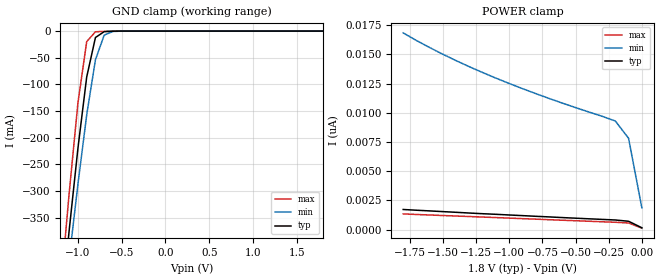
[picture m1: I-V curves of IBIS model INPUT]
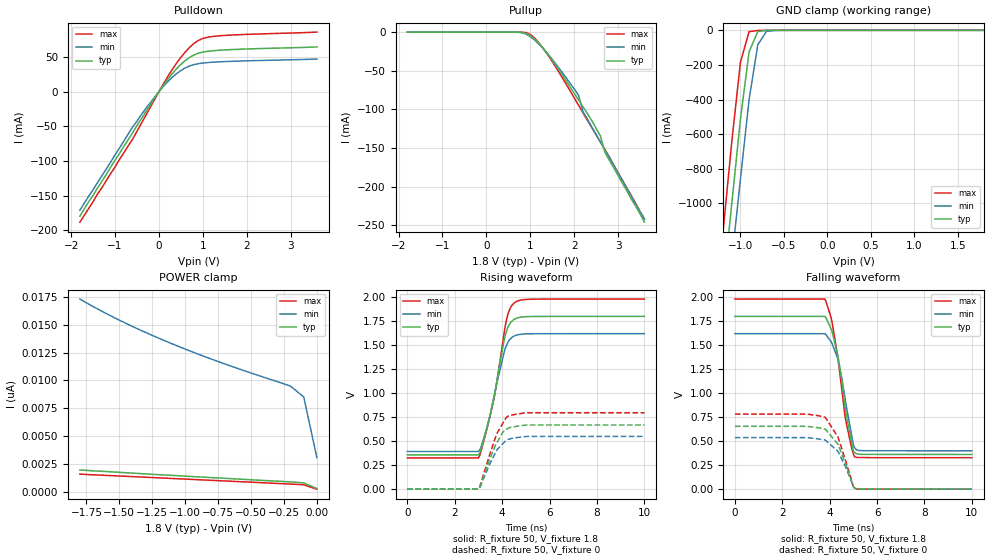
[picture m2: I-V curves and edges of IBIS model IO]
|   PERICOM SEMICONDUCTOR CORP
|   IBIS Model of PI4ULS3V204
|   Product Family: ULS
|   TSSOP-14 (L) Package
[IBIS Ver] 3.2
[Comment char] |_char
[File Name] pi4uls3v204_l_18v.ibs
[File Rev] 1.0
[Source] File originated at Pericom Semiconductor Corp.
[Date] 09/06/2017
[Disclaimer] (C) Copyright PERICOM Semiconductor Corporation
   All rights reserved
  Pericom Semiconductor Corporation hereby grants the user of
  this IBIS model a non-exclusive, nontransferable license to
  use this IBIS model under the following terms.
  This IBIS model is provided on an "AS IS" basis and Pericom
  makes absolutely no warranty with respect to the information
  contained herein. PERICOM DISCLAIMS AND CUSTOMER WAIVES ALL
  WARRANTIES, EXPRESSED OR IMPLIED, INCLUDING WARRANTIES OF
  MERCHANTABILITY OR FITNESS FOR A PARTICULAR PURPOSE. The
  entire risk as to quality and performance is with the customer.
  Accordingly, in no event shall the company be liable for any
  damages, whether in contract or tort, including any lost
  profits or other incidental, consequential, exemplary, or
  punitive damages arising out of the use or application of the
  IBIS model provided in this package. Further, Pericom reserves
  the right to make changes without notice to any product herein
  to improve reliability, function, or design. Pericom does not
  convey any license under patent rights or any other intellectual
  property rights, including those of third parties.
  The user is granted this license only to use the IBIS model
  and is not granted rights to sell, load, rent, lease or license
  the IBIS model in whole or in part, or in modified form to anyone
  other than user. User may modify the IBIS model to suit its specific
  application but rights to derivative works and such modifications
  shall belong to Pericom.
  Pericom is not obligated to provide maintenance or support
  for the licensed IBIS model.
  Contact Pericom at ATTN: APPLICATION ENGINEERING / IBIS MODELS
  1545 Barber Lane Milpitas, CA 95035 USA.
[Component] PI4ULS3V204
[Manufacturer] Pericom Semiconductor Corp.
[Package]
| variable   typ   min   max
R_pkg   0.04200   0.03995   0.04405
L_pkg   2.30669n   2.21200n   2.40138n
C_pkg   0.21108p   0.20715p   0.21500p
[Pin] signal_name  model_name   R_pin   L_pin   C_pin
1   VCCA   POWER   0.03604  2.91900n  0.20300p
2   A1   IO   0.03631  2.73467n  0.19100p
3   A2   IO   0.03658  2.55033n  0.17900p
4   A3   IO   0.03686  2.36600n  0.16700p
5   A4   IO   0.03658  2.55033n  0.17900p
6   NC   NC   0.03631  2.73467n  0.19100p
7   GND   GND   0.03604  2.91900n  0.20300p
8   EN   INPUT   0.03604  2.91900n  0.20300p
9   NC   NC   0.03631  2.73467n  0.19100p
10   B4   IO   0.03658  2.55033n  0.17900p
11   B3   IO   0.03686  2.36600n  0.16700p
12   B2   IO   0.03658  2.55033n  0.17900p
13   B1   IO   0.03631  2.73467n  0.19100p
14   VCCB   POWER   0.03604  2.91900n  0.20300p
| Models and submodels in the file (2): INPUT (Input), IO (I/O)
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[Model] INPUT
Model_type Input
Vinl = 540mV
Vinh = 1.26V
| variable   typ   min   max
C_comp   0.220pF   0.210pF   0.230pF
[Voltage Range]   1.8000V   1.6200V   1.9800V
[POWER Clamp Reference] 1.8000V   1.6200V   1.9800V
[GND Clamp Reference]   0.0000V   0.0000V   0.0000V
[Temperature Range]   25   85   -40
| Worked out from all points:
|   GND clamp passes 1 mA (typ) near -0.70 V on its own axis
[GND Clamp]
| Voltage   I(typ)   I(min)   I(max)
-1.8V     -1.564A    -1.492A    -1.669A
-1.2V     -536.3mA   -573.9mA   -488.8mA
-1.1V     -373.8mA   -427.8mA   -304mA
-1V       -219.8mA   -287.2mA   -134.4mA
-900mV    -86.22mA   -157.4mA   -19.74mA
-800mV    -12.06mA   -53.77mA   -1.311mA
-700mV    -1.032mA   -7.522mA   -526.9uA
-600mV    -210.6uA   -734.5uA   -129.9uA
1.8V      68.64pA    148.9pA    67.17pA
[POWER Clamp]
| Voltage   I(typ)   I(min)   I(max)
-1.8V     1.724nA    16.84nA    1.345nA
-1.5V     1.541nA    15.01nA    1.207nA
-1.3V     1.419nA    13.94nA    1.121nA
-1.1V     1.31nA     12.97nA    1.031nA
-700mV    1.089nA    11.23nA    849pA
-200mV    824.2pA    9.299nA    628.2pA
-100mV    715.1pA    7.823nA    568pA
0V        162pA      1.877nA    124.8pA
[Model]   IO
Model_type I/O
Vinl=0.15
Vinh=1.65
Enable   Active-High
Vref =   1.8
Rref =   50
Cref =   15p
Vmeas =   0.9
| variable   typ   min   max
C_comp   3.740E-12   3.730E-12   3.750E-12
[Voltage Range]   1.8000V   1.6200V   1.9800V
[POWER Clamp Reference] 1.8000V   1.6200V   1.9800V
[GND Clamp Reference]   0.000E+00   0.000E+00   0.000E+00
[Pullup Reference]   1.8000V   1.6200V   1.9800V
[Pulldown Reference]   0.000E+00   0.000E+00   0.000E+00
[Temperature Range]   25   85   -40
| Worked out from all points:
|   slope of the pulldown table from 0 to 0.27 V, typ, clamps not added: 11.5 ohm
|   slope of the pullup table from 0 to 0.27 V, typ, clamps not added: 10.1 kohm
|   GND clamp passes 1 mA (typ) near -0.71 V on its own axis
|   rising waveform, R_fixture 50, V_fixture 1.8: 20-80 % time 685ps typ, 688ps min, 709ps max; typ from 0.358 V to 1.8 V
|   falling waveform, R_fixture 50, V_fixture 1.8: 20-80 % time 570ps typ, 551ps min, 567ps max; typ from 1.8 V to 0.362 V
|   rising waveform, R_fixture 50, V_fixture 0: 20-80 % time 672ps typ, 677ps min, 690ps max; typ from 0.002 V to 0.669 V
|   falling waveform, R_fixture 50, V_fixture 0: 20-80 % time 697ps typ, 685ps min, 708ps max; typ from 0.656 V to 0.002 V
[GND Clamp]
| Voltage   I(typ)   I(min)   I(max)
-1.8V     -4.449A    -4.635A    -4.26A
-1.2V     -1.497A    -1.804A    -1.164A
-1.1V     -1.005A    -1.332A    -648.2mA
-1V       -514.4mA   -860.5mA   -184.8mA
-900mV    -123.7mA   -400mA     -7.522mA
-800mV    -6.738mA   -83.76mA   -632.8uA
-700mV    -436.7uA   -5.934mA   -74.67uA
-500mV    -2.716uA   -28.54uA   -128.4nA
1.8V      284.4pA    9.393nA    26.33pA
[POWER Clamp]
| Voltage   I(typ)   I(min)   I(max)
-1.8V     1.954nA    17.31nA    1.574nA
-1.5V     1.737nA    15.41nA    1.408nA
-1.3V     1.594nA    14.3nA     1.297nA
-1.1V     1.466nA    13.29nA    1.184nA
-700mV    1.201nA    11.48nA    964.7pA
-200mV    880.2pA    9.489nA    684.2pA
-100mV    794.6pA    8.509nA    622.1pA
0V        284.4pA    3.048nA    225.7pA
[Pullup]
| Voltage   I(typ)   I(min)   I(max)
-1.8V     8.38uA     5.146uA    14.63uA
700mV     -77.1uA    -122.1uA   -69.61uA
900mV     -1.314mA   -2.344mA   -505.3uA
1V        -4.356mA   -5.707mA   -2.879mA
1.2V      -14.84mA   -15.61mA   -14.06mA
1.4V      -28.66mA   -28.16mA   -29.49mA
1.7V      -52.77mA   -49.99mA   -56.17mA
2.1V      -87.81mA   -81.6mA    -94.49mA
2.2V      -96.54mA   -102.8mA   -104.2mA
2.6V      -134.5mA   -142.7mA   -142.2mA
2.7V      -155.5mA   -152.1mA   -151.9mA
3.6V      -246mA     -242.2mA   -241.7mA
[Pulldown]
| Voltage   I(typ)   I(min)   I(max)
-1.8V     -180mA     -171.1mA   -188.5mA
-1.6V     -159.1mA   -151mA     -168.8mA
-600mV    -59.62mA   -51.1mA    -68.72mA
-100mV    -9.784mA   -8.125mA   -11.61mA
200mV     17.7mA     14.26mA    21.55mA
400mV     32.89mA    25.86mA    40.89mA
600mV     44.87mA    34.26mA    57.2mA
800mV     53.05mA    39.13mA    69.66mA
1V        57.15mA    41.32mA    76.77mA
1.3V      59.48mA    42.83mA    80.2mA
3.6V      64.62mA    47.1mA     86.04mA
[Rising Waveform]
R_fixture = 50
V_fixture = 1.8
V_fixture_min = 1.62
V_fixture_max = 1.98
| Time   V(typ)   V(min)   V(max)
0s        358.2mV    394mV      326.6mV
3ns       358.1mV    393.9mV    326.6mV
3.1ns     412.2mV    437.3mV    390.1mV
3.3ns     583.9mV    597.4mV    574.2mV
3.65ns    951.5mV    960.9mV    940.5mV
4.1ns     1.576V     1.444V     1.659V
4.25ns    1.692V     1.534V     1.831V
4.55ns    1.774V     1.6V       1.947V
5.2ns     1.798V     1.619V     1.978V
10ns      1.8V       1.62V      1.98V
[Falling Waveform]
R_fixture = 50
V_fixture = 1.8
V_fixture_min = 1.62
V_fixture_max = 1.98
| Time   V(typ)   V(min)   V(max)
0s        1.8V       1.62V      1.98V
3.8ns     1.799V     1.619V     1.979V
4.1ns     1.642V     1.518V     1.742V
4.35ns    1.388V     1.353V     1.364V
4.5ns     1.149V     1.172V     1.06V
4.65ns    856mV      944.3mV    755.9mV
5ns       396.8mV    463.4mV    365.6mV
5.05ns    385.9mV    433.5mV    339.4mV
5.4ns     363.7mV    402.3mV    330.9mV
10ns      362.4mV    400.9mV    328.9mV
[Rising Waveform]
R_fixture = 50
V_fixture = 0
V_fixture_min = 0
V_fixture_max = 0
| Time   V(typ)   V(min)   V(max)
0s        1.563mV    1.642mV    1.482mV
3ns       1.563mV    1.641mV    1.482mV
3.1ns     51.73mV    40.85mV    60.55mV
3.45ns    294.8mV    246.6mV    342.8mV
3.75ns    473.5mV    396.4mV    562.4mV
4.05ns    601.7mV    480.3mV    696.7mV
4.2ns     627.1mV    516.8mV    754.9mV
4.35ns    644mV      526mV      769.7mV
5.1ns     669.5mV    550.5mV    797mV
10ns      669.4mV    550.5mV    796.8mV
[Falling Waveform]
R_fixture = 50
V_fixture = 0
V_fixture_min = 0
V_fixture_max = 0
| Time   V(typ)   V(min)   V(max)
0s        655.7mV    538.1mV    782.8mV
3ns       655.6mV    538mV      782.7mV
3.8ns     627.3mV    513.4mV    751.6mV
4.35ns    468.5mV    394.7mV    543.7mV
4.7ns     246.1mV    216mV      275.6mV
5ns       28.07mV    28.74mV    27.39mV
5.05ns    18.52mV    12.69mV    7.515mV
5.15ns    4.836mV    3.192mV    2.892mV
5.3ns     2.083mV    2.19mV     1.846mV
10ns      1.576mV    1.659mV    1.492mV
[Ramp]
| variable   typ   min   max
dV/dt_r   4.0082E-01/6.7203E-10  3.2938E-01/6.7780E-10  4.7728E-01/6.9062E-10
dV/dt_f   8.6256E-01/5.7028E-10  7.3146E-01/5.5107E-10  9.9060E-01/5.6692E-10
R_load = 50
